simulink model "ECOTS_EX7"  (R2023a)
settings: Solver=ode23tb  StartTime=0.0  StopTime=meas.Time(end)  RelTol=1e-3
libraries: component_lib x38, slpidlib x3

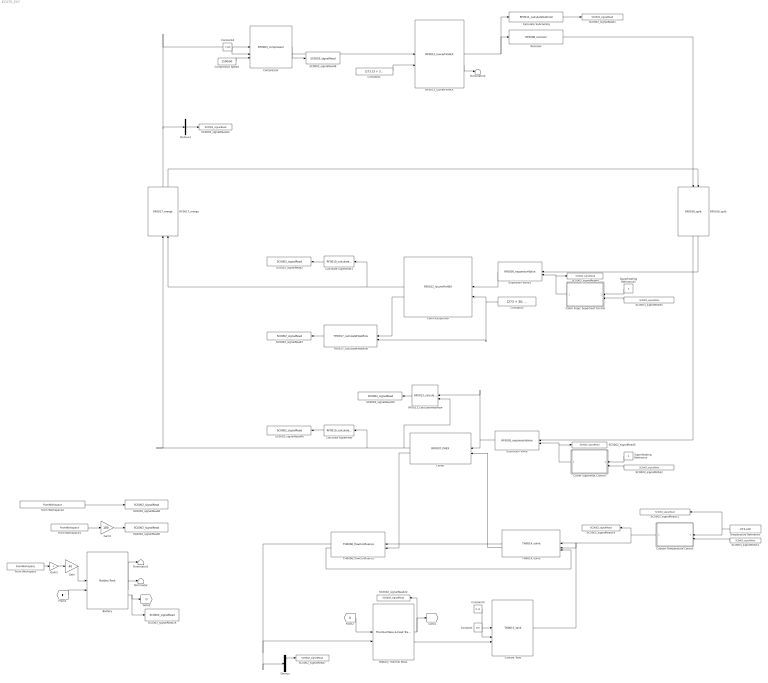
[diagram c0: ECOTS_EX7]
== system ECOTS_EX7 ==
  Battery : component_lib/Battery Pack  SOC_0=1  Nx=40  Ny=180
  Battery Thermal Mass : component_lib/Thermal Mass & Heat Transfer  n=100  d=10e-3  L=4  m=40 * 180 * 0.048  cp=1040  T_0=273 + 20
  Cabin Evap. Superheat Control : Subsystem
  Cabin Evaporator : component_lib/Thermal Systems/RF0012_louverFinHEX  N_tub=30  T_L=0.4  T_p=10.15e-3  T_d=16e-3  N_ch=18  a=1.3e-3  b=0.58e-3  L_a=23  F_p=1.4e-3  L_p=1.7e-3  L_l=6.4e-3  H=8.15e-3  d_f=16e-3  F_d=16e-3  N_nod=10
  Calculate Subcooling : component_lib/Thermal Systems/RF0011_calculateSubCool
  Calculate Superheat : component_lib/Thermal Systems/RF0010_calculateSuperHeat
  Calculate Superheat1 : component_lib/Thermal Systems/RF0010_calculateSuperHeat
  Chiller : component_lib/Thermal Systems/RF0007_PHEX  N_ch=10  L=180e-3  B=65e-3  H=2e-3  t=0.3e-3  D_h=2.61e-3  N_nod=10
  Chiller Superheat Control : Subsystem
  Compressor : component_lib/Thermal Systems/RF0003_compressor  V_disp=0.00017  N_ref=2000
  Compressor Speed : Constant  Value=1500/60
  Constant : Constant  Value=2e5
  Constant1 : Constant  Value=[273.15 + 35; 1e5; 8]
  Constant2 : Constant  Value=[273 + 30; 1e5; 0.4]
  Constant3 : Constant  Value=0.15
  Constant4 : Constant  Value=1.5e6
  Coolant Tank : component_lib/Thermal Systems/TH0013_tank  V=5e-3  T0=273.15 + 20
  Coolant Temperature Control : Subsystem
  Demux : Demux  Outputs=3
  Demux1 : Demux  Outputs=3
  Expansion Valve : component_lib/Thermal Systems/RF0005_expansionValve  D=3.5*1.8e-3  p_min=100e3
  Expansion Valve1 : component_lib/Thermal Systems/RF0005_expansionValve  D=3.5*1.8e-3  p_min=100e3
  From Workspace : FromWorkspace  VariableName=[meas.Time, meas.Current]
  From Workspace1 : FromWorkspace  VariableName=[meas.Time, meas.Voltage]
  From Workspace2 : FromWorkspace  VariableName=[meas.Time, meas.Battery_Temp_degC + 273.15]
  Gain : Gain  Gain=40
  Gain1 : Gain  Gain=180
  Gain2 : Gain  Gain=-1
  RF0012_louverFinHEX : component_lib/Thermal Systems/RF0012_louverFinHEX  N_tub=80  T_L=0.95  T_p=10.15e-3  T_d=16e-3  N_ch=18  a=1.3e-3  b=0.58e-3  L_a=23  F_p=1.4e-3  L_p=1.7e-3  L_l=6.4e-3  H=8.15e-3  d_f=16e-3  F_d=16e-3  N_nod=10
  RF0013_calculateHeatflow : component_lib/Thermal Systems/RF0013_calculateHeatflow
  RF0016_split : component_lib/Thermal Systems/RF0016_split
  RF0017_merge : component_lib/Thermal Systems/RF0017_merge  V=1e-3
  Receiver : component_lib/Thermal Systems/RF0008_receiver  V=100e-3  h0=280e3  p0=1.5e6  p_gain=1e4
  SC0002_signalRead1 : component_lib/Data & Control/SC0002_signalRead  SigName=condenserSubCooling
  SC0002_signalRead10 : component_lib/Data & Control/SC0002_signalRead  SigName=chillerCooling
  SC0002_signalRead11 : component_lib/Data & Control/SC0002_signalRead  SigName=evaporatorPressure
  SC0002_signalRead14 : component_lib/Data & Control/SC0002_signalRead  SigName=generatedHeat
  SC0002_signalRead19 : component_lib/Data & Control/SC0002_signalRead  SigName=chillerBypassValve
  SC0002_signalRead2 : component_lib/Data & Control/SC0002_signalRead  SigName=cabinEvaporatorSuperheat
  SC0002_signalRead21 : component_lib/Data & Control/SC0002_signalRead  SigName=coolantTemperatureReference
  SC0002_signalRead22 : component_lib/Data & Control/SC0002_signalRead  SigName=batteryTemperature
  SC0002_signalRead3 : component_lib/Data & Control/SC0002_signalRead  SigName=airConditioningLoad
  SC0002_signalRead4 : component_lib/Data & Control/SC0002_signalRead  SigName=cabinExpansionValve
  SC0002_signalRead40 : component_lib/Data & Control/SC0002_signalRead  SigName=chillerSuperheat
  SC0002_signalRead5 : component_lib/Data & Control/SC0002_signalRead  SigName=chillerExpansionValve
  SC0002_signalRead6 : component_lib/Data & Control/SC0002_signalRead  SigName=measuredBatteryVoltage
  SC0002_signalRead7 : component_lib/Data & Control/SC0002_signalRead  SigName=coolantTemperature
  SC0002_signalRead8 : component_lib/Data & Control/SC0002_signalRead  SigName=measuredBatteryTemperature
  SC0002_signalRead9 : component_lib/Data & Control/SC0002_signalRead  SigName=compressorPower
  SC0003_signalWrite2 : component_lib/Data & Control/SC0003_signalWrite  SigName=chillerSuperheat
  SC0003_signalWrite3 : component_lib/Data & Control/SC0003_signalWrite  SigName=coolantTemperature
  SC0003_signalWrite5 : component_lib/Data & Control/SC0003_signalWrite  SigName=cabinEvaporatorSuperheat
  Superheating Reference : Constant  Value=5
  Superheating Reference1 : Constant  Value=5
  TH0006_flowConfluence : component_lib/Thermal Systems/TH0006_flowConfluence  gain=0.01
  TH0014_valve : component_lib/Thermal Systems/TH0014_valve  d=10e-2  dr=5e-2  C_d=0.9
  TH0017_calculateHeatflow : component_lib/Thermal Systems/TH0017_calculateHeatflow
  Temperature Reference : Constant  Value=273+20
  Terminator : Terminator
  Terminator1 : Terminator
  Terminator2 : Terminator
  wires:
  Calculate Superheat/1 -> SC0002_signalRead40/1
  Compressor Speed/1 -> Compressor/3
  Compressor/2 -> SC0002_signalRead9/1
  RF0012_louverFinHEX/1 -> Calculate Subcooling/1, Receiver/1
  Chiller Superheat Control/1(EXV [-]) -> Expansion Valve/2, SC0002_signalRead5/1
  Calculate Subcooling/1 -> SC0002_signalRead1/1
  Superheating Reference/1 -> Chiller Superheat Control/1(T_ref [K])
  SC0003_signalWrite2/1 -> Chiller Superheat Control/2(T_sup [K])
  [Q] -> Battery Thermal Mass/1
  Battery Thermal Mass/1 -> [T], SC0002_signalRead22/1
  Constant3/1 -> Coolant Tank/1
  Constant/1 -> Coolant Tank/2
  Battery Thermal Mass/2 -> Coolant Tank/3
  TH0014_valve/2 -> Chiller/2
  TH0014_valve/1 -> TH0006_flowConfluence/1
  Chiller/2 -> TH0006_flowConfluence/2
  TH0006_flowConfluence/2 -> TH0014_valve/3
  Coolant Tank/1 -> TH0014_valve/2
  Coolant Temperature Control/1(cv [-]) -> TH0014_valve/1, SC0002_signalRead19/1
  Temperature Reference/1 -> Coolant Temperature Control/1(T_ref [K]), SC0002_signalRead21/1
  SC0003_signalWrite3/1 -> Coolant Temperature Control/2(T [K])
  Constant1/1 -> RF0012_louverFinHEX/2
  RF0012_louverFinHEX/2 -> Terminator2/1
  Receiver/1 -> RF0016_split/1
  Superheating Reference1/1 -> Cabin Evap. Superheat Control/1(T_ref [K])
  SC0003_signalWrite5/1 -> Cabin Evap. Superheat Control/2(T_sup [K])
  RF0016_split/1 -> Expansion Valve/1
  RF0017_merge/1 -> Compressor/1, Demux1/1
  Expansion Valve1/1 -> Cabin Evaporator/1
  RF0016_split/2 -> Expansion Valve1/1
  Compressor/1 -> RF0012_louverFinHEX/1
  Cabin Evaporator/1 -> Calculate Superheat1/1, RF0017_merge/2
  Calculate Superheat1/1 -> SC0002_signalRead2/1
  Constant2/1 -> TH0017_calculateHeatflow/2, Cabin Evaporator/2
  TH0017_calculateHeatflow/1 -> SC0002_signalRead3/1
  Cabin Evaporator/2 -> TH0017_calculateHeatflow/1
  Cabin Evap. Superheat Control/1(EXV [-]) -> Expansion Valve1/2, SC0002_signalRead4/1
  Demux/1 -> SC0002_signalRead7/1
  TH0006_flowConfluence/1 -> Battery Thermal Mass/2, Demux/1
  Battery/1 -> Terminator1/1
  Gain/1 -> Battery/1
  Battery/2 -> Terminator/1
  [T] -> Battery/2
  From Workspace2/1 -> SC0002_signalRead8/1
  Gain2/1 -> Gain/1
  Battery/3 -> SC0002_signalRead14/1, [Q]
  Gain1/1 -> SC0002_signalRead6/1
  From Workspace1/1 -> Gain1/1
  From Workspace/1 -> Gain2/1
  Constant4/1 -> Compressor/2
  RF0017_merge/2 -> RF0016_split/2
  RF0013_calculateHeatflow/1 -> SC0002_signalRead10/1
  Expansion Valve/1 -> RF0013_calculateHeatflow/1, Chiller/1
  Chiller/1 -> RF0017_merge/1, Calculate Superheat/1, RF0013_calculateHeatflow/2
  Demux1/2 -> SC0002_signalRead11/1

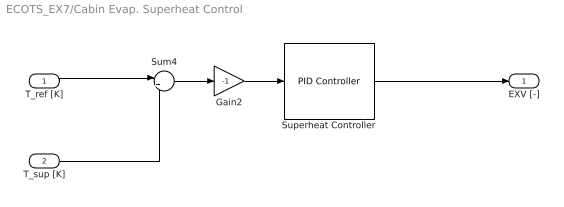
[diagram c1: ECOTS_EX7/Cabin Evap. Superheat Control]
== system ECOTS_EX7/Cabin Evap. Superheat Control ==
  T_ref [K] : Inport
  T_sup [K] : Inport  Port=2
  Gain2 : Gain  Gain=-1
  Sum4 : Sum  Inputs=|+-
  Superheat Controller : slpidlib/PID Controller  Controller=PI  Form=Parallel  TimeDomain=Continuous-time  UseExternalTs=off  SampleTime=-1  IntegratorMethod=Forward Euler  FilterMethod=Forward Euler  ControllerParametersSource=internal  P=1e-2  I=1e-2  UseKiTs=off  D=0  N=100  UseFilter=on  TunerSelectOption=Transfer Function Based (PID Tuner App)  InitialConditionSource=internal  InitialConditionForIntegrator=0.2  InitialConditionForFilter=0  DifferentiatorICPrevScaledInput=0  ExternalReset=none  TrackingMode=off  Kt=1  LimitOutput=on  SatLimitsSource=internal  UpperSaturationLimit=0.999  LowerSaturationLimit=0.001  LinearizeAsGain=on  AntiWindupMode=back-calculation  Kb=1  LimitIntegrator=off  UpperIntegratorSaturationLimit=inf  LowerIntegratorSaturationLimit=-inf  POutMin=[]  POutMax=[]  IOutMin=[]  IOutMax=[]  DOutMin=[]  DOutMax=[]  NOutMin=[]  NOutMax=[]  SumOutMin=[]  SumOutMax=[]  SaturationOutMin=[]  SaturationOutMax=[]  PParamMin=[]  PParamMax=[]  IParamMin=[]  IParamMax=[]  DParamMin=[]  DParamMax=[]  NParamMin=[]  NParamMax=[]  KbParamMin=[]  KbParamMax=[]  KtParamMin=[]  KtParamMax=[]  KbOutMin=[]  KbOutMax=[]  KtOutMin=[]  KtOutMax=[]  IntegratorOutMin=[]  IntegratorOutMax=[]  FilterOutMin=[]  FilterOutMax=[]  SumI1OutMin=[]  SumI1OutMax=[]  SumI2OutMin=[]  SumI2OutMax=[]  SumI3OutMin=[]  SumI3OutMax=[]  SumI4OutMin=[]  SumI4OutMax=[]  SumDOutMin=[]  SumDOutMax=[]  DifferentiatorOutMin=[]  DifferentiatorOutMax=[]  FilterDiffOutCoefMin=[]  FilterDiffOutCoefMax=[]  ReciprocalOutMin=[]  ReciprocalOutMax=[]  SumDenOutMin=[]  SumDenOutMax=[]  SumNumOutMin=[]  SumNumOutMax=[]  DivideOutMin=[]  DivideOutMax=[]  UdiffTsProdOutMin=[]  UdiffTsProdOutMax=[]  NTsProdOutMin=[]  NTsProdOutMax=[]  UintegralTsProdOutMin=[]  UintegralTsProdOutMax=[]  UngainTsProdOutMin=[]  UngainTsProdOutMax=[]  ClampingZeroOutDataTypeStr=Inherit: Inherit via back propagation  ClampingZeroOutMin=[]  ClampingZeroOutMax=[]  FilterDenConstantOutDataTypeStr=Inherit: Inherit via back propagation  FilterDenConstantOutMin=[]  FilterDenConstantOutMax=[]  PCopyOutDataTypeStr=Inherit: Inherit via back propagation  PCopyOutMin=[]  PCopyOutMax=[]  NCopyOutDataTypeStr=Inherit: Inherit via back propagation  NCopyOutMin=[]  NCopyOutMax=[]  IntegratorContinuousStateAttributes=''  IntegratorStateMustResolveToSignalObject=off  IntegratorRTWStateStorageClass=Auto  FilterContinuousStateAttributes=''  FilterStateMustResolveToSignalObject=off  FilterRTWStateStorageClass=Auto  ParallelPVariant=InternalParameters  IdealPVariant=Disabled  IVariant=InternalParameters  DVariant=Disabled  IntegratorVariant=Continuous  SatVariant=Enabled  AWVariant=BackCalculation  PCopyVariant=Disabled  TRVariant=Disabled  FdbkBlocksVariant=Forward  IdealPFdbkVariant=Disabled  SatFdbkVariant=Disabled  DerivativeFilterVariant=Disabled  NVariant=Disabled  NCopyVariant=Disabled_SignalSpec  FilterICVariant=Disabled  IntegratorICVariant=InternalICs  ExternalResetVariant=Disabled  TRSumVariant=Passthrough  SumFdbkVariant=Disabled  SumVariant=Sum_PI  TsampFilterVariant=InternalTs  TsampNgainVariant=Passthrough  TsampIntegralVariant=Disabled_SignalSpec  ExternalSaturationOutDataTypeStr=Inherit: Same as second input
  EXV [-] : Outport
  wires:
  Sum4/1 -> Gain2/1
  T_ref [K]/1 -> Sum4/1
  T_sup [K]/1 -> Sum4/2
  Gain2/1 -> Superheat Controller/1
  Superheat Controller/1 -> EXV [-]/1

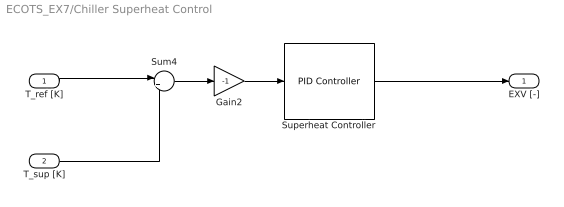
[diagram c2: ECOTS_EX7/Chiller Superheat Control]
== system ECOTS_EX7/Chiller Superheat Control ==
  T_ref [K] : Inport
  T_sup [K] : Inport  Port=2
  Gain2 : Gain  Gain=-1
  Sum4 : Sum  Inputs=|+-
  Superheat Controller : slpidlib/PID Controller  Controller=PI  Form=Parallel  TimeDomain=Continuous-time  UseExternalTs=off  SampleTime=-1  IntegratorMethod=Forward Euler  FilterMethod=Forward Euler  ControllerParametersSource=internal  P=1e-2  I=1e-2  UseKiTs=off  D=0  N=100  UseFilter=on  TunerSelectOption=Transfer Function Based (PID Tuner App)  InitialConditionSource=internal  InitialConditionForIntegrator=0.2  InitialConditionForFilter=0  DifferentiatorICPrevScaledInput=0  ExternalReset=none  TrackingMode=off  Kt=1  LimitOutput=on  SatLimitsSource=internal  UpperSaturationLimit=0.999  LowerSaturationLimit=0.001  LinearizeAsGain=on  AntiWindupMode=back-calculation  Kb=1  LimitIntegrator=off  UpperIntegratorSaturationLimit=inf  LowerIntegratorSaturationLimit=-inf  POutMin=[]  POutMax=[]  IOutMin=[]  IOutMax=[]  DOutMin=[]  DOutMax=[]  NOutMin=[]  NOutMax=[]  SumOutMin=[]  SumOutMax=[]  SaturationOutMin=[]  SaturationOutMax=[]  PParamMin=[]  PParamMax=[]  IParamMin=[]  IParamMax=[]  DParamMin=[]  DParamMax=[]  NParamMin=[]  NParamMax=[]  KbParamMin=[]  KbParamMax=[]  KtParamMin=[]  KtParamMax=[]  KbOutMin=[]  KbOutMax=[]  KtOutMin=[]  KtOutMax=[]  IntegratorOutMin=[]  IntegratorOutMax=[]  FilterOutMin=[]  FilterOutMax=[]  SumI1OutMin=[]  SumI1OutMax=[]  SumI2OutMin=[]  SumI2OutMax=[]  SumI3OutMin=[]  SumI3OutMax=[]  SumI4OutMin=[]  SumI4OutMax=[]  SumDOutMin=[]  SumDOutMax=[]  DifferentiatorOutMin=[]  DifferentiatorOutMax=[]  FilterDiffOutCoefMin=[]  FilterDiffOutCoefMax=[]  ReciprocalOutMin=[]  ReciprocalOutMax=[]  SumDenOutMin=[]  SumDenOutMax=[]  SumNumOutMin=[]  SumNumOutMax=[]  DivideOutMin=[]  DivideOutMax=[]  UdiffTsProdOutMin=[]  UdiffTsProdOutMax=[]  NTsProdOutMin=[]  NTsProdOutMax=[]  UintegralTsProdOutMin=[]  UintegralTsProdOutMax=[]  UngainTsProdOutMin=[]  UngainTsProdOutMax=[]  ClampingZeroOutDataTypeStr=Inherit: Inherit via back propagation  ClampingZeroOutMin=[]  ClampingZeroOutMax=[]  FilterDenConstantOutDataTypeStr=Inherit: Inherit via back propagation  FilterDenConstantOutMin=[]  FilterDenConstantOutMax=[]  PCopyOutDataTypeStr=Inherit: Inherit via back propagation  PCopyOutMin=[]  PCopyOutMax=[]  NCopyOutDataTypeStr=Inherit: Inherit via back propagation  NCopyOutMin=[]  NCopyOutMax=[]  IntegratorContinuousStateAttributes=''  IntegratorStateMustResolveToSignalObject=off  IntegratorRTWStateStorageClass=Auto  FilterContinuousStateAttributes=''  FilterStateMustResolveToSignalObject=off  FilterRTWStateStorageClass=Auto  ParallelPVariant=InternalParameters  IdealPVariant=Disabled  IVariant=InternalParameters  DVariant=Disabled  IntegratorVariant=Continuous  SatVariant=Enabled  AWVariant=BackCalculation  PCopyVariant=Disabled  TRVariant=Disabled  FdbkBlocksVariant=Forward  IdealPFdbkVariant=Disabled  SatFdbkVariant=Disabled  DerivativeFilterVariant=Disabled  NVariant=Disabled  NCopyVariant=Disabled_SignalSpec  FilterICVariant=Disabled  IntegratorICVariant=InternalICs  ExternalResetVariant=Disabled  TRSumVariant=Passthrough  SumFdbkVariant=Disabled  SumVariant=Sum_PI  TsampFilterVariant=InternalTs  TsampNgainVariant=Passthrough  TsampIntegralVariant=Disabled_SignalSpec  ExternalSaturationOutDataTypeStr=Inherit: Same as second input
  EXV [-] : Outport
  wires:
  Sum4/1 -> Gain2/1
  T_ref [K]/1 -> Sum4/1
  T_sup [K]/1 -> Sum4/2
  Gain2/1 -> Superheat Controller/1
  Superheat Controller/1 -> EXV [-]/1

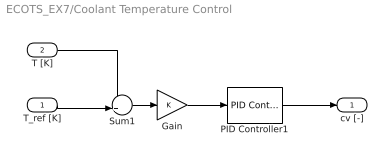
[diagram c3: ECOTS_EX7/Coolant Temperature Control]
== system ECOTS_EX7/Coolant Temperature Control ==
  T_ref [K] : Inport
  T [K] : Inport  Port=2
  Gain : Gain
  PID Controller1 : slpidlib/PID Controller  Controller=PI  Form=Parallel  TimeDomain=Continuous-time  UseExternalTs=off  SampleTime=-1  IntegratorMethod=Forward Euler  FilterMethod=Forward Euler  ControllerParametersSource=internal  P=1e-1  I=1e-3  UseKiTs=off  D=0  N=100  UseFilter=on  TunerSelectOption=Transfer Function Based (PID Tuner App)  ZeroCross=off  InitialConditionSource=internal  InitialConditionForIntegrator=0.5  InitialConditionForFilter=0.5  DifferentiatorICPrevScaledInput=0  ExternalReset=none  TrackingMode=off  Kt=1  LimitOutput=on  SatLimitsSource=internal  UpperSaturationLimit=0.95  LowerSaturationLimit=0.05  LinearizeAsGain=on  AntiWindupMode=back-calculation  Kb=1  LimitIntegrator=off  UpperIntegratorSaturationLimit=inf  LowerIntegratorSaturationLimit=-inf  POutMin=[]  POutMax=[]  IOutMin=[]  IOutMax=[]  DOutMin=[]  DOutMax=[]  NOutMin=[]  NOutMax=[]  SumOutMin=[]  SumOutMax=[]  SaturationOutMin=[]  SaturationOutMax=[]  PParamMin=[]  PParamMax=[]  IParamMin=[]  IParamMax=[]  DParamMin=[]  DParamMax=[]  NParamMin=[]  NParamMax=[]  KbParamMin=[]  KbParamMax=[]  KtParamMin=[]  KtParamMax=[]  KbOutMin=[]  KbOutMax=[]  KtOutMin=[]  KtOutMax=[]  IntegratorOutMin=[]  IntegratorOutMax=[]  FilterOutMin=[]  FilterOutMax=[]  SumI1OutMin=[]  SumI1OutMax=[]  SumI2OutMin=[]  SumI2OutMax=[]  SumI3OutMin=[]  SumI3OutMax=[]  SumI4OutMin=[]  SumI4OutMax=[]  SumDOutMin=[]  SumDOutMax=[]  DifferentiatorOutMin=[]  DifferentiatorOutMax=[]  FilterDiffOutCoefMin=[]  FilterDiffOutCoefMax=[]  ReciprocalOutMin=[]  ReciprocalOutMax=[]  SumDenOutMin=[]  SumDenOutMax=[]  SumNumOutMin=[]  SumNumOutMax=[]  DivideOutMin=[]  DivideOutMax=[]  UdiffTsProdOutMin=[]  UdiffTsProdOutMax=[]  NTsProdOutMin=[]  NTsProdOutMax=[]  UintegralTsProdOutMin=[]  UintegralTsProdOutMax=[]  UngainTsProdOutMin=[]  UngainTsProdOutMax=[]  ClampingZeroOutDataTypeStr=Inherit: Inherit via back propagation  ClampingZeroOutMin=[]  ClampingZeroOutMax=[]  FilterDenConstantOutDataTypeStr=Inherit: Inherit via back propagation  FilterDenConstantOutMin=[]  FilterDenConstantOutMax=[]  PCopyOutDataTypeStr=Inherit: Inherit via back propagation  PCopyOutMin=[]  PCopyOutMax=[]  NCopyOutDataTypeStr=Inherit: Inherit via back propagation  NCopyOutMin=[]  NCopyOutMax=[]  IntegratorContinuousStateAttributes=''  IntegratorStateMustResolveToSignalObject=off  IntegratorRTWStateStorageClass=Auto  FilterContinuousStateAttributes=''  FilterStateMustResolveToSignalObject=off  FilterRTWStateStorageClass=Auto  ParallelPVariant=InternalParameters  IdealPVariant=Disabled  IVariant=InternalParameters  DVariant=Disabled  IntegratorVariant=Continuous  SatVariant=Enabled  AWVariant=BackCalculation  PCopyVariant=Disabled  TRVariant=Disabled  FdbkBlocksVariant=Forward  IdealPFdbkVariant=Disabled  SatFdbkVariant=Disabled  DerivativeFilterVariant=Disabled  NVariant=Disabled  NCopyVariant=Disabled_SignalSpec  FilterICVariant=Disabled  IntegratorICVariant=InternalICs  ExternalResetVariant=Disabled  TRSumVariant=Passthrough  SumFdbkVariant=Disabled  SumVariant=Sum_PI  TsampFilterVariant=InternalTs  TsampNgainVariant=Passthrough  TsampIntegralVariant=Disabled_SignalSpec  ExternalSaturationOutDataTypeStr=Inherit: Same as second input
  Sum1 : Sum  Inputs=-+|
  cv [-] : Outport
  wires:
  T [K]/1 -> Sum1/1
  Gain/1 -> PID Controller1/1
  Sum1/1 -> Gain/1
  PID Controller1/1 -> cv [-]/1
  T_ref [K]/1 -> Sum1/2
